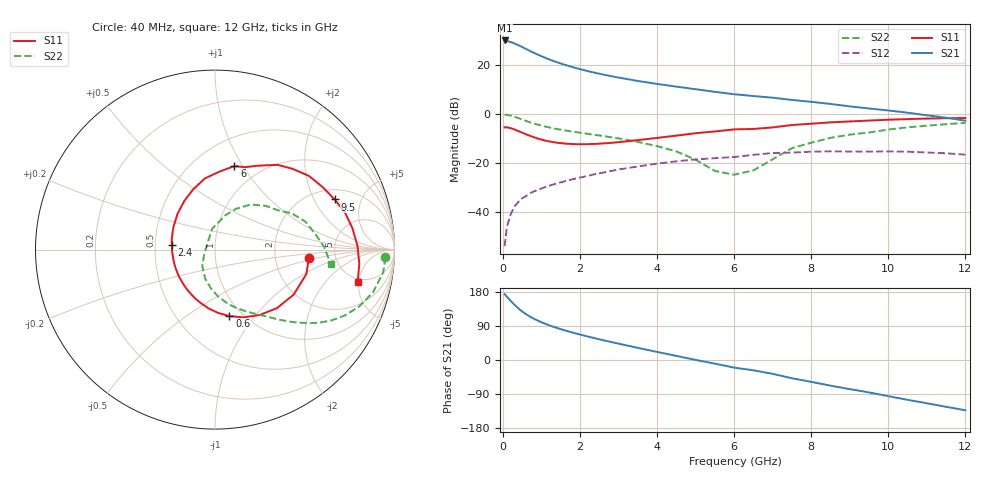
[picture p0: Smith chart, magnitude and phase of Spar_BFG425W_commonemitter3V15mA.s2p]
! Filename: 315bfg425.001
! BFG425W Field C1
! V1=8.465E-001V,V2=3.000E+000V, I1=1.942E-004A, I2=1.497E-002A
# GHz  S  MA  R 50
!  S11  S21  S12  S22
!Freq(GHz)  Mag  Ang  Mag  Ang  Mag  Ang  Mag  Ang
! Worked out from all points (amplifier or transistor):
!   44 points, 40 MHz to 12 GHz, reference 50 ohm
!   highest |S21| = 29.8 dB at 40 MHz (marker M1)
!   |S21| within 3 dB of that: start of sweep to 535.4 MHz
!   unconditionally stable (mu >= 1): 1.588 GHz to end of sweep
!   at 700 MHz: K = 0.65, MSG = 29.0 dB, |S12| = -32.4 dB
!   at 2.4 GHz: K = 1.13, MAG = 18.4 dB, |S12| = -24.6 dB
!   at 12 GHz: K = 1.36, MAG = 3.3 dB, |S12| = -16.7 dB
!   S11 on the Smith chart (normalised r, x): 40 MHz: 3.15, -0.41; 600 MHz: 0.87, -0.75; 2.4 GHz: 0.61, +0.03; 6 GHz: 0.76, +0.92; 9.5 GHz: 2.53, +2.96; 12 GHz: 4.49, -4.83
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0.04  0.525 -5.1  30.97 174.0  0.002 63.1  0.95 -2.6
0.1  0.527 -15.0  30.17 167.1  0.005 82.1  0.946 -7.6
0.2  0.505 -29.8  28.76 155.6  0.009 75.6  0.912 -15.1
0.3  0.475 -43.3  26.82 145.4  0.013 70.9  0.863 -21.6
0.4  0.441 -55.8  24.73 136.1  0.016 67.3  0.81 -27.0
0.5  0.409 -67.5  22.65 127.7  0.019 63.8  0.758 -31.4
0.6  0.379 -77.7  20.66 120.7  0.021 61.6  0.71 -35.0
0.8  0.331 -95.7  17.32 109.0  0.026 58.2  0.629 -40.4
0.9  0.311 -103.6  15.95 104.0  0.028 57.2  0.598 -42.6
1  0.296 -111.1  14.73 99.5  0.03 56.3  0.57 -44.5
1.2  0.272 -124.5  12.72 91.5  0.034 54.7  0.524 -47.9
1.6  0.246 -148.3  9.903 78.3  0.042 52.2  0.456 -53.8
2.2  0.239 -177.1  7.356 62.0  0.054 47.3  0.388 -62.8
2.4  0.242 174.4  6.764 57.0  0.059 45.5  0.368 -65.9
3.5  0.289 136.2  4.637 32.0  0.084 32.6  0.266 -85.4
4.5  0.357 110.0  3.55 10.8  0.107 18.5  0.17 -108.8
6  0.478 76.9  2.488 -20.1  0.131 -5.6  0.057 135.6
6.5  0.488 70.2  2.284 -27.2  0.145 -8.6  0.07 118.9
8.5  0.665 38.2  1.576 -67.8  0.171 -45.6  0.321 51.5
9.5  0.723 22.7  1.274 -85.6  0.169 -62.3  0.414 31.9
10.5  0.775 8.8  1.047 -105.1  0.168 -81.0  0.527 17.2
12  0.815 -12.8  0.719 -132.7  0.146 -111.1  0.65 -7.3
